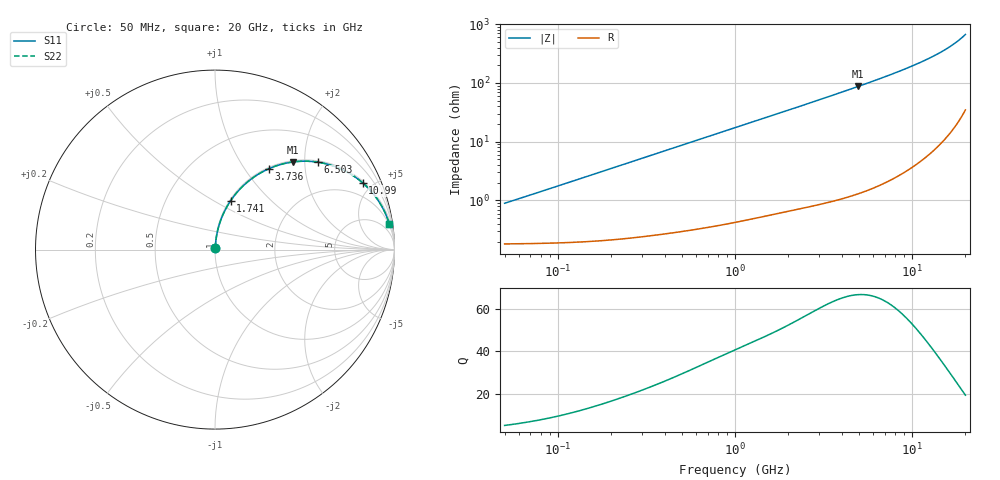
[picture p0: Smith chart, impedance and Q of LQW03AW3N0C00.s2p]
!Murata Part Number: LQW03AW3N0C00
!These Parameters are Measured in Series Mode Connection
!  o--[Z]--o
!Port1  Port2
!  o-------o
!Freq. Start=50[MHz] Stop=20[GHz], 401[Steps]
# Hz S RI R 50
!Freq.(Hz) S11(Real) S11(Imag) S21(Real) S21(Imag) S12(Real) S12(Imag) S22(Real) S22(Imag)
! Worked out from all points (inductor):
!   401 points, 50 MHz to 20 GHz, reference 50 ohm
!   read as one part in series: L = 2.79 nH near 51.52 MHz
!   highest Q = 67 at 4.967 GHz (marker M1), where L = 2.79 nH
!   S11 on the Smith chart (normalised r, x): 50 MHz: 1.00, +0.02; 1.741 GHz: 1.01, +0.60; 3.736 GHz: 1.02, +1.29; 6.503 GHz: 1.04, +2.33; 10.99 GHz: 1.09, +4.38; 20 GHz: 2, +13
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5e7  0.0019 0.00875  0.9981 -0.00875  0.9981 -0.00875  0.0019 0.00875
1.364002e8  0.00254 0.0238  0.9975 -0.0238  0.9975 -0.0238  0.00254 0.0238
2.33884e8  0.00388 0.0406  0.9961 -0.0406  0.9961 -0.0406  0.00388 0.0406
3.721004e8  0.00675 0.0641  0.9932 -0.0641  0.9932 -0.0641  0.00675 0.0641
6.285508e8  0.0149 0.1069  0.9851 -0.1069  0.9851 -0.1069  0.0149 0.1069
1e9  0.0327 0.1661  0.9673 -0.1661  0.9673 -0.1661  0.0327 0.1661
1.349283e9  0.0555 0.2182  0.9445 -0.2182  0.9445 -0.2182  0.0555 0.2182
1.740566e9  0.0868 0.2717  0.9132 -0.2717  0.9132 -0.2717  0.0868 0.2717
2.211938e9  0.1309 0.3283  0.8691 -0.3283  0.8691 -0.3283  0.1309 0.3283
2.728004e9  0.185 0.3799  0.815 -0.3799  0.815 -0.3799  0.185 0.3799
3.168813e9  0.2339 0.4153  0.7661 -0.4153  0.7661 -0.4153  0.2339 0.4153
3.736399e9  0.2983 0.4498  0.7017 -0.4498  0.7017 -0.4498  0.2983 0.4498
4.966507e9  0.4326 0.488  0.5674 -0.488  0.5674 -0.488  0.4326 0.488
5.683258e9  0.5032 0.4926  0.4968 -0.4926  0.4968 -0.4926  0.5032 0.4926
6.503449e9  0.5751 0.4867  0.4249 -0.4867  0.4249 -0.4867  0.5751 0.4867
7.442007e9  0.6459 0.4703  0.3541 -0.4703  0.3541 -0.4703  0.6459 0.4703
8.907419e9  0.7341 0.4332  0.2659 -0.4332  0.2659 -0.4332  0.7341 0.4332
1.098561e10  0.8226 0.372  0.1774 -0.372  0.1774 -0.372  0.8226 0.372
1.314879e10  0.8834 0.3089  0.1166 -0.3089  0.1166 -0.3089  0.8834 0.3089
1.527346e10  0.9231 0.2518  0.0769 -0.2518  0.0769 -0.2518  0.9231 0.2518
1.721783e10  0.9479 0.2045  0.0521 -0.2045  0.0521 -0.2045  0.9479 0.2045
2e10  0.9708 0.1444  0.0292 -0.1444  0.0292 -0.1444  0.9708 0.1444
